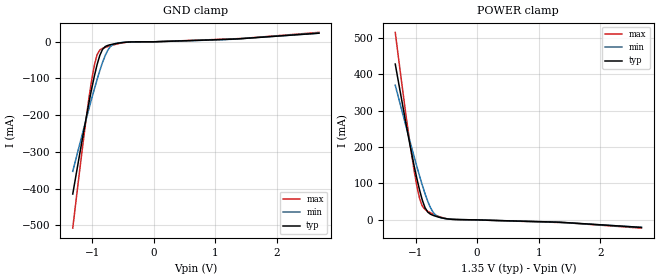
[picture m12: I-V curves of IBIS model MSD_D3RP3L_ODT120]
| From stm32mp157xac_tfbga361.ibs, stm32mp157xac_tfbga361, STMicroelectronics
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[Model] MSD_D3RP3L_ODT120
Model_type   Input
C_comp 2.197pF   2.122pF   2.281pF
Vinh = 810.000mV
Vinl = 540.000mV
[Temperature Range]   25.000   125.000   -40.000
[Voltage Range]   1.350V   1.283V   1.450V
[GND Clamp Reference]   0.00V   0.00V   0.00V
[POWER Clamp Reference]   1.350V   1.283V   1.450V
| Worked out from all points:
|   GND clamp passes 1 mA (typ) near -0.44 V on its own axis
|   POWER clamp passes 1 mA (typ) near -0.33 V on its own axis
[GND Clamp]
-1.318V   -415mA     -353.2mA   -508mA
-1.142V   -246.2mA   -238.2mA   -264.1mA
-1.011V   -128.1mA   -154.9mA   -104.3mA
-966.7mV  -92.99mA   -128.4mA   -63.5mA
-922.7mV  -62.07mA   -102.8mA   -35.06mA
-878.8mV  -37.14mA   -78.64mA   -22.4mA
-834.9mV  -20.69mA   -56.51mA   -18.03mA
-747mV    -9.66mA    -22.26mA   -13mA
-659.1mV  -6.198mA   -6.845mA   -8.626mA
-571.2mV  -3.566mA   -2.927mA   -4.866mA
1.274V    7.314mA    6.947mA    8.003mA
2.68V     23.44mA    23.63mA    25.7mA
[Power Clamp]
-1.33V    427.4mA    369.4mA    514.3mA
-1.155V   263mA      256mA      286mA
-1.023V   147.8mA    172.9mA    134.9mA
-934.9mV  81.61mA    120.2mA    58.32mA
-890.9mV  54.31mA    95.28mA    38.09mA
-847mV    33.56mA    72.06mA    28.73mA
-803mV    21.38mA    51.24mA    23.61mA
-715.1mV  12.36mA    20.81mA    15.87mA
-627.3mV  7.666mA    8.056mA    9.573mA
-539.4mV  4.249mA    4.099mA    4.84mA
1.438V    -7.433mA   -7.9mA     -7.783mA
2.668V    -20.7mA    -20.53mA   -22.68mA
